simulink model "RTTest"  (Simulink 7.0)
settings: Solver=FixedStepDiscrete  StartTime=0.0  StopTime=inf  RelTol=1e-3
PreLoadFcn:
  | initialize;
  | scramInitialize;
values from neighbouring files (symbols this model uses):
  controlPeriod = 1/2048    (= 0.00048828125)    [initialize.m]
  nAcc = size(ra, 2)    [initialize.m]
  nAct = self.nAct    [animation.m]    (also in initialize.m = size(rh, 2))
  nAdcU = 6    [initialize.m]
  node = scgtnodestruct(node)    [scramInitialize.m]
  x = []    [loadbin.m]    (also in quake.m = 365; viewer.m = 40; player.m = xPanel + panelWide + margin; resondemo.m = xOrigin + marginWide + panelWide + plotMarginWide)
undefined symbols (not defined in the file or in its folder): DiscIntNeverNeededParam
libraries: cwcec_scgtLib x3, xpclib x2

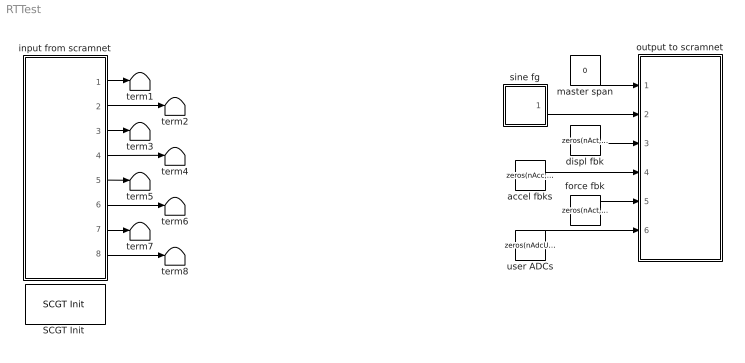
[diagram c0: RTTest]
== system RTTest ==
  "SCGT Init " : cwcec_scgtLib/SCGT Init   node=node  pci=-1
  accel fbks : Constant  Value=zeros(nAcc, 1)  OutDataType=sfix(16)  OutScaling=2^0
  displ fbk : Constant  Value=zeros(nAct, 1)  OutDataType=sfix(16)  OutScaling=2^0
  force fbk : Constant  Value=zeros(nAct, 1)  OutDataType=sfix(16)  OutScaling=2^0
  input from scramnet : Subsystem
  master span : Constant  Value=0  OutDataType=sfix(16)  OutScaling=2^0
  output to scramnet : Subsystem
  sine fg : Subsystem  mask(Sine Function Generator){id=x, ampl=0.3, freq=4, phase=0, spanInterval=1, samplePeriod=controlPeriod}
      mask prompts: id "DOF"; ampl "Amplitude"; freq "Frequency (Hz)"; phase "Phase (deg)"; spanInterval "Span interval (sec)"; samplePeriod "Sample period (sec)"
  term{1..8} (8 alike) : Terminator
  user ADCs : Constant  Value=zeros(nAdcU, 1)  OutDataType=sfix(16)  OutScaling=2^0
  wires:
  user ADCs/1 -> output to scramnet/6(user adcs)
  master span/1 -> output to scramnet/1(master span)
  sine fg/1(out) -> output to scramnet/2(ref)
  input from scramnet/1(master span) -> term1/1
  input from scramnet/3(displ fbk) -> term3/1
  input from scramnet/4(veloc fbk) -> term4/1
  input from scramnet/6(force fbk) -> term6/1
  input from scramnet/8(user adcs) -> term8/1
  input from scramnet/2(ref) -> term2/1
  input from scramnet/5(accel fbk) -> term5/1
  displ fbk/1 -> output to scramnet/3(displ fbk)
  accel fbks/1 -> output to scramnet/4(accel fbks)
  force fbk/1 -> output to scramnet/5(force fbk)
  input from scramnet/7(valve cmd) -> term7/1

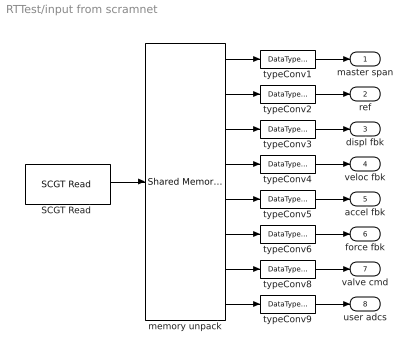
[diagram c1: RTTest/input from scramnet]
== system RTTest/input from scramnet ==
  "SCGT Read " : cwcec_scgtLib/SCGT Read   partition=node.Partitions(7:14)  ts=controlPeriod  pci=-1
  memory unpack : xpclib/Shared Memory/Shared Memory Unpack   partition=node.Partitions(7:14)
  typeConv{1..6,8..9} (8 alike) : DataTypeConversion  OutDataTypeMode=double  OutDataType=sfix(16)  OutScaling=2^0
  master span : Outport  OutDataType=sfix(16)  OutScaling=2^0
  ref : Outport  Port=2  OutDataType=sfix(16)  OutScaling=2^0
  displ fbk : Outport  Port=3  OutDataType=sfix(16)  OutScaling=2^0
  veloc fbk : Outport  Port=4  OutDataType=sfix(16)  OutScaling=2^0
  accel fbk : Outport  Port=5  OutDataType=sfix(16)  OutScaling=2^0
  force fbk : Outport  Port=6  OutDataType=sfix(16)  OutScaling=2^0
  valve cmd : Outport  Port=7  OutDataType=sfix(16)  OutScaling=2^0
  user adcs : Outport  Port=8  OutDataType=sfix(16)  OutScaling=2^0
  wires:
  memory unpack/6 -> typeConv6/1
  memory unpack/5 -> typeConv5/1
  memory unpack/4 -> typeConv4/1
  memory unpack/3 -> typeConv3/1
  memory unpack/7 -> typeConv8/1
  memory unpack/2 -> typeConv2/1
  memory unpack/8 -> typeConv9/1
  memory unpack/1 -> typeConv1/1
  typeConv9/1 -> user adcs/1
  typeConv8/1 -> valve cmd/1
  typeConv6/1 -> force fbk/1
  typeConv5/1 -> accel fbk/1
  typeConv4/1 -> veloc fbk/1
  typeConv3/1 -> displ fbk/1
  typeConv2/1 -> ref/1
  typeConv1/1 -> master span/1
  "SCGT Read "/1 -> memory unpack/1

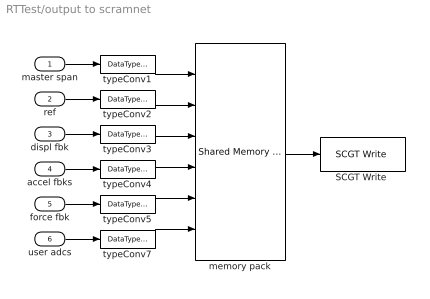
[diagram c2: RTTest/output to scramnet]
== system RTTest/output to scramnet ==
  master span : Inport  OutDataType=sfix(16)  OutScaling=2^0
  ref : Inport  Port=2  OutDataType=sfix(16)  OutScaling=2^0
  displ fbk : Inport  Port=3  OutDataType=sfix(16)  OutScaling=2^0
  accel fbks : Inport  Port=4  OutDataType=sfix(16)  OutScaling=2^0
  force fbk : Inport  Port=5  OutDataType=sfix(16)  OutScaling=2^0
  user adcs : Inport  Port=6  OutDataType=sfix(16)  OutScaling=2^0
  "SCGT Write " : cwcec_scgtLib/SCGT Write   partition=node.Partitions(1:6)  ts=controlPeriod  pci=-1
  memory pack : xpclib/Shared Memory/Shared Memory Pack   partition=node.Partitions(1:6)
  typeConv{1..5,7} (6 alike) : DataTypeConversion  OutDataTypeMode=single  OutDataType=sfix(16)  OutScaling=2^0
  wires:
  typeConv7/1 -> memory pack/6
  typeConv5/1 -> memory pack/5
  user adcs/1 -> typeConv7/1
  force fbk/1 -> typeConv5/1
  typeConv4/1 -> memory pack/4
  typeConv3/1 -> memory pack/3
  typeConv2/1 -> memory pack/2
  typeConv1/1 -> memory pack/1
  memory pack/1 -> "SCGT Write "/1
  accel fbks/1 -> typeConv4/1
  displ fbk/1 -> typeConv3/1
  ref/1 -> typeConv2/1
  master span/1 -> typeConv1/1

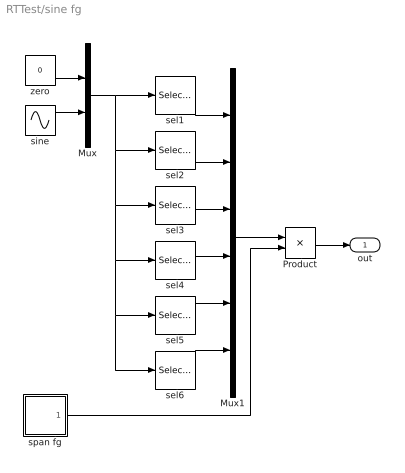
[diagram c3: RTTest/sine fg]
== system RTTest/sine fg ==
  Mux : Mux  Inputs=2
  Mux1 : Mux  Inputs=6
  Product : Product  OutDataType=sfix(16)  OutScaling=2^0
  sel1 : Selector  InputPortWidth=2  IndexOptions=Index vector (dialog)  Indices=(id==1)+1  OutputSizes=1
  sel2 : Selector  InputPortWidth=2  IndexOptions=Index vector (dialog)  Indices=(id==2)+1  OutputSizes=1
  sel3 : Selector  InputPortWidth=2  IndexOptions=Index vector (dialog)  Indices=(id==3)+1  OutputSizes=1
  sel4 : Selector  InputPortWidth=2  IndexOptions=Index vector (dialog)  Indices=(id==4)+1  OutputSizes=1
  sel5 : Selector  InputPortWidth=2  IndexOptions=Index vector (dialog)  Indices=(id==5)+1  OutputSizes=1
  sel6 : Selector  InputPortWidth=2  IndexOptions=Index vector (dialog)  Indices=(id==6)+1  OutputSizes=1
  sine : Sin  Amplitude=ampl  Frequency=2 * pi * freq  Phase=phase*180/pi  SampleTime=samplePeriod
  span fg : Subsystem  mask{spanInterval=spanInterval, samplePeriod=samplePeriod}
      mask prompts: spanInterval "Span interval (sec)"; samplePeriod "Sample period (sec)"
  zero : Constant  Value=0  OutDataType=sfix(16)  OutScaling=2^0  SampleTime=samplePeriod
  out : Outport  OutDataType=sfix(16)  OutScaling=2^0
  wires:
  Mux/1 -> sel1/1, sel6/1, sel5/1, sel4/1, sel3/1, sel2/1
  sel6/1 -> Mux1/6
  sel5/1 -> Mux1/5
  sel4/1 -> Mux1/4
  sel3/1 -> Mux1/3
  sel2/1 -> Mux1/2
  sel1/1 -> Mux1/1
  sine/1 -> Mux/2
  zero/1 -> Mux/1
  Mux1/1 -> Product/1
  Product/1 -> out/1
  span fg/1(out) -> Product/2

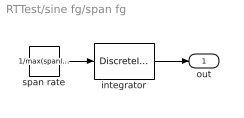
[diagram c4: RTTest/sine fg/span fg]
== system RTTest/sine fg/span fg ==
  integrator : DiscreteIntegrator  SampleTime=samplePeriod  OutDataType=sfix(16)  OutScaling=2^0  LimitOutput=on  UpperSaturationLimit=1  LowerSaturationLimit=0  ICPrevOutput=DiscIntNeverNeededParam  ICPrevScaledInput=DiscIntNeverNeededParam
  span rate : Constant  Value=1/max(spanInterval,samplePeriod)  OutDataType=sfix(16)  OutScaling=2^0  SampleTime=samplePeriod
  out : Outport  OutDataType=sfix(16)  OutScaling=2^0
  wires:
  integrator/1 -> out/1
  span rate/1 -> integrator/1
